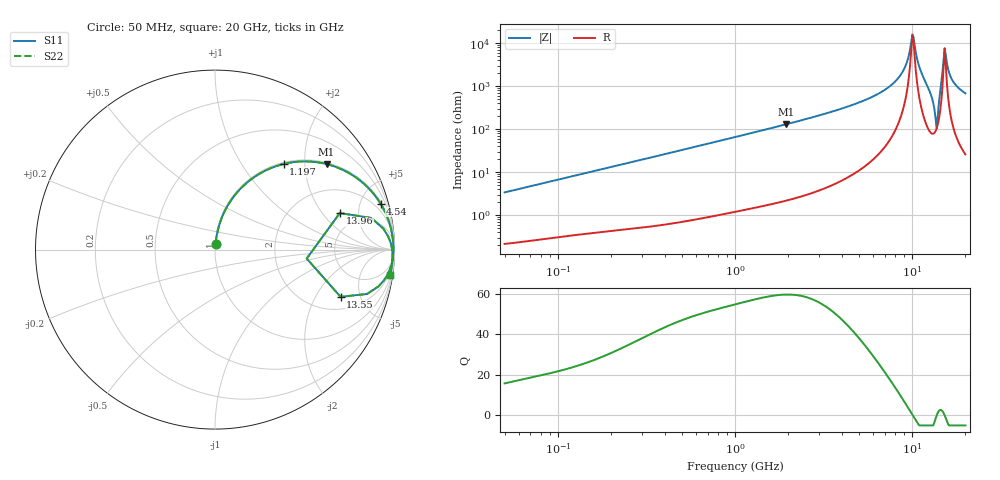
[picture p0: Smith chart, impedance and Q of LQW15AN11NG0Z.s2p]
!Murata Part Number: LQW15AN11NG0Z
!These Parameters are Measured in Series Mode Connection
!  o--[Z]--o
!Port1  Port2
!  o-------o
!Freq. Start=50[MHz] Stop=20[GHz], 401[Steps]
# Hz S RI R 50
!Freq.(Hz) S11(Real) S11(Imag) S21(Real) S21(Imag) S12(Real) S12(Imag) S22(Real) S22(Imag)
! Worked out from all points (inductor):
!   401 points, 50 MHz to 20 GHz, reference 50 ohm
!   read as one part in series: L = 10.7 nH near 51.52 MHz
!   highest Q = 59.5 at 1.933 GHz (marker M1), where L = 10.6 nH
!   self-resonance near 10.04 GHz
!   S11 on the Smith chart (normalised r, x): 50 MHz: 1.00, +0.07; 1.197 GHz: 1.03, +1.57; 4.54 GHz: 1.17, +7.14; 13.55 GHz: 2.77, -3.30; 13.96 GHz: 3.54, +3.03; 20 GHz: 2, -14
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5e7  0.00328 0.0336  0.9967 -0.0336  0.9967 -0.0336  0.00328 0.0336
1.364002e8  0.0116 0.0889  0.9884 -0.0889  0.9884 -0.0889  0.0116 0.0889
3.721004e8  0.0606 0.2271  0.9394 -0.2271  0.9394 -0.2271  0.0606 0.2271
1e9  0.3021 0.4501  0.6979 -0.4501  0.6979 -0.4501  0.3021 0.4501
1.196911e9  0.3821 0.4771  0.6179 -0.4771  0.6179 -0.4771  0.3821 0.4771
1.932977e9  0.6215 0.4767  0.3785 -0.4767  0.3785 -0.4767  0.6215 0.4767
2.728004e9  0.7749 0.409  0.2251 -0.409  0.2251 -0.409  0.7749 0.409
4.539627e9  0.9221 0.2564  0.0779 -0.2564  0.0779 -0.2564  0.9221 0.2564
7.442007e9  0.984 0.1006  0.016 -0.1006  0.016 -0.1006  0.984 0.1006
8.907419e9  0.9924 0.0431  0.00761 -0.0431  0.00761 -0.0431  0.9924 0.0431
1.004137e10  0.9939 0.00164  0.00606 -0.00164  0.00606 -0.00164  0.9939 0.00164
1.034674e10  0.9937 -0.00968  0.00633 0.00968  0.00633 0.00968  0.9937 -0.00968
1.115139e10  0.9912 -0.0415  0.00882 0.0415  0.00882 0.0415  0.9912 -0.0415
1.257102e10  0.9682 -0.1259  0.0318 0.1259  0.0318 0.1259  0.9682 -0.1259
1.314879e10  0.9107 -0.2054  0.0893 0.2054  0.0893 0.2054  0.9107 -0.2054
1.354865e10  0.6997 -0.2631  0.3003 0.2631  0.3003 0.2631  0.6997 -0.2631
1.396067e10  0.6952 0.2035  0.3048 -0.2035  0.3048 -0.2035  0.6952 0.2035
1.438523e10  0.938 0.117  0.062 -0.117  0.062 -0.117  0.938 0.117
1.504638e10  0.9837 0.0186  0.0163 -0.0186  0.0163 -0.0186  0.9837 0.0186
1.550395e10  0.9886 -0.0149  0.0114 0.0149  0.0114 0.0149  0.9886 -0.0149
1.696185e10  0.9875 -0.0738  0.0125 0.0738  0.0125 0.0738  0.9875 -0.0738
2e10  0.9737 -0.1421  0.0263 0.1421  0.0263 0.1421  0.9737 -0.1421
